PROGRAM RegistrationMarkSimulation
VAR_INPUT
	ProductLength 					: LREAL;
END_VAR
VAR_OUTPUT
	RegistrationSignal 				: BOOL;
END_VAR
VAR_IN_OUT
	Axis 							: AXIS_REF;
END_VAR
VAR
	RegistrationPosition			: LREAL;
	initialized						: BOOL;
	Variation						: LREAL;
	random							: DRAND;
END_VAR

(*
	Simulation of a registration mark for each product.
	The signal is randomly modified to simulate a registration deviation.
 *)

IF NOT initialized THEN
	RegistrationPosition := Axis.NcToPlc.SetPos;
	initialized := TRUE;
END_IF

IF Axis.NcToPlc.SetPos > RegistrationPosition + ProductLength + Variation THEN
	random();
	Variation := random.Num  * 2 - 1; (* registration error simulation *)
	RegistrationSignal := TRUE;
	RegistrationPosition := Axis.NcToPlc.SetPos;
ELSIF Axis.NcToPlc.SetPos > (RegistrationPosition + ProductLength/10.0) THEN
	RegistrationSignal := FALSE;
END_IF

END_PROGRAM
